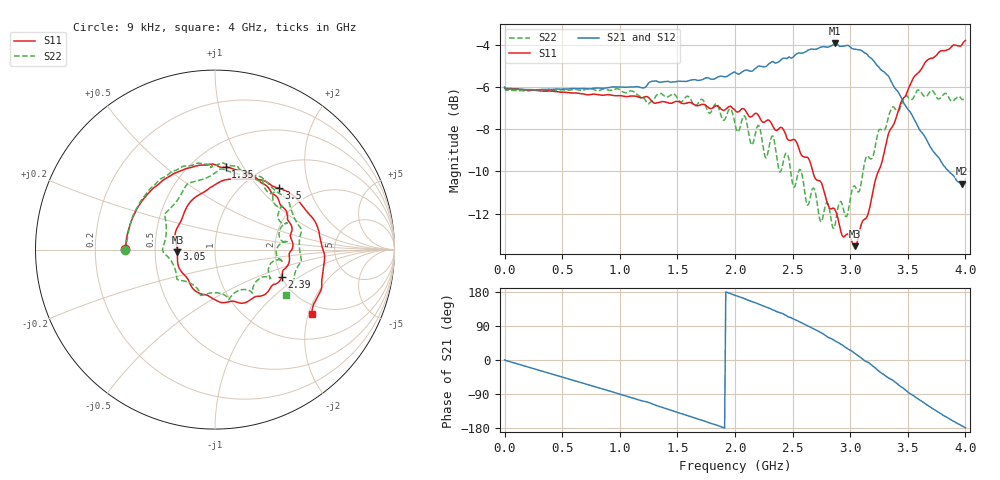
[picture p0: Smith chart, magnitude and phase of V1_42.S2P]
! ZVRE, 3.40
! symbol freq-unit parameter-type data-format keyword impedance-ohm
#  HZ  S  RI  R  50
! freq  reS11  imS11  reS21  imS21  reS12  imS12  reS22  imS22
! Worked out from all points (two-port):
!   401 points, 9 kHz to 4 GHz, reference 50 ohm
!   highest |S21| = -3.91 dB at 2.87 GHz (marker M1); lowest = -10.6 dB at 3.97 GHz (marker M2)
!   |S21| within 3 dB of the highest: start of sweep to 3.485 GHz
!   lowest |S11| = -13.6 dB at 3.04 GHz (marker M3), VSWR 1.53, Z = 32.7 - j0.993 ohm
!   |S11| at or under -10 dB: 2.675 GHz to 3.244 GHz (568.5 MHz wide, 19.2 % of centre)
!   |S22| runs from -12.7 to -6.0 dB; largest |S21 - S12| = 0.023
!   S11 on the Smith chart (normalised r, x): 9 kHz: 0.33, +0.00; 1.35 GHz: 0.72, +0.84; 2.39 GHz: 2.02, -0.72; 3.05 GHz: 0.65, +0.00; 3.5 GHz: 1.42, +1.29; 4 GHz: 1.69, -2.10
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9000  -0.5 0.00129  0.5021 0.00134  0.502 -0.00143  -0.5003 -0.000275
3.300083e8  -0.4545 0.1856  0.4313 -0.2444  0.4366 -0.2423  -0.4547 0.1934
6.700075e8  -0.3397 0.3447  0.2478 -0.4317  0.2541 -0.431  -0.3352 0.3609
9.800068e8  -0.1795 0.4439  0.015 -0.502  0.0191 -0.5053  -0.1764 0.4652
1.340006e9  0.0542 0.4584  -0.2746 -0.4363  -0.2737 -0.4417  0.0369 0.4826
1.350006e9  0.0597 0.4583  -0.2812 -0.4317  -0.2802 -0.4364  0.0401 0.4827
1.740005e9  0.2976 0.3449  -0.5003 -0.1647  -0.5015 -0.1708  0.2681 0.3699
2.000004e9  0.4043 0.1788  -0.5373 0.0891  -0.5396 0.083  0.3547 0.2075
2.200004e9  0.4313 0.00677  -0.4778 0.2971  -0.4834 0.2919  0.4052 0.0405
2.390004e9  0.373 -0.15  -0.3303 0.4759  -0.3401 0.4729  0.301 -0.0927
2.460003e9  0.3191 -0.1994  -0.243 0.5368  -0.2556 0.5344  0.3047 -0.1625
2.670003e9  0.1263 -0.2941  0.0647 0.6145  0.0554 0.6208  0.0791 -0.2757
2.870003e9  -0.106 -0.2329  0.4086 0.4891  0.4 0.4964  -0.1545 -0.1797
3.040002e9  -0.2096 -0.0145  0.5891 0.1862  0.5888 0.1933  -0.2919 0.0058
3.050002e9  -0.2111 0.00239  0.5954 0.1644  0.5973 0.1678  -0.2884 0.0182
3.160002e9  -0.1827 0.1755  0.5896 -0.0708  0.5947 -0.0734  -0.275 0.2038
3.340001e9  0.0602 0.3892  0.3502 -0.396  0.3554 -0.3963  0.00985 0.4339
3.500001e9  0.3552 0.3425  0.0442 -0.4425  0.0556 -0.4511  0.28 0.3847
3.700001e9  0.5797 0.0984  -0.2072 -0.2949  -0.21 -0.3021  0.4782 0.1176
3.8e9  0.6095 -0.0632  -0.2681 -0.192  -0.2746 -0.1937  0.4776 -0.0355
3.97e9  0.5435 -0.3246  -0.2941 -0.0319  -0.2991 -0.0258  0.4177 -0.2134
4e9  0.5382 -0.361  -0.2971 -0.00566  -0.2975 -0.00213  0.3971 -0.2502
